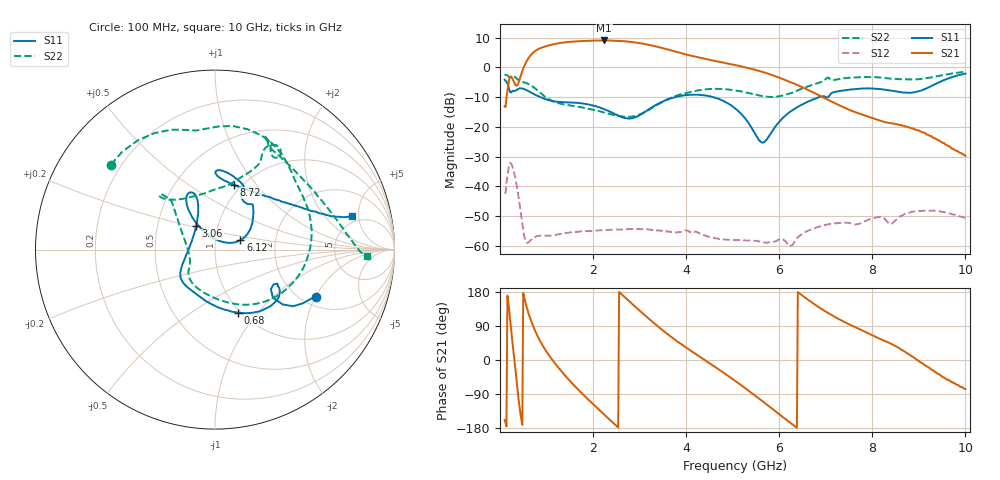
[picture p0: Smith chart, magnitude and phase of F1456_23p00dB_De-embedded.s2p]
! Integrated Device Technology
! Corporate Headquarters
! 6024 Silver Creek Valley Road
! San Jose, CA 95138  USA
! Phone:  1-408-284-8200
! Toll Free:  1-800-223-1366
! Webpage:  http://www.idt.com/
! Timing and RF Division
! 515 Groton Road, Suite 102
! Westford, MA 01886-6024
! Device:  F1456
! Description: 6-bit 0.5 dB Transmit Variable Gain Amplifier
! Frequency:  2100.0 -  2950.00 MHz
! Package:  6x6 mm Thin QFN Plastic Package: 28 pin
! State:  46
! Atten State:  23.0 dB
! Voltage:  +5.00 Volts
! Current:  216.983 mA
! Data:  The device was measured on a the F1455 evaluation board which has
!  individual transmission lines to the RF pins.  Data was collected
!  using a calibrated network analyzer.  The evaluation board was
!  de-embedded using a TRL calibration technique.
!  The reference plane is the edge of the package pin.
!  Pin  1 = CSb
!  Pin  2 = DATA
!  Pin  3 = CLK
!  Pin  4 = RSET
!  Pin  5 = GND
!  Pin  6 = RFIN  = Port 1
!  Pin  7 = GND
!  Pin  8 = NC
!  Pin  9 = NC
!  Pin 10 = NC
!  Pin 11 = NC
!  Pin 12 = NC
!  Pin 13 = NC
!  Pin 14 = /STBY
!  Pin 15 = GND
!  Pin 16 = RFOUT  = Port 2
!  Pin 17 = GND
!  Pin 18 = NC
!  Pin 19 = NC
!  Pin 20 = NC
!  Pin 21 = GND
!  Pin 22 = NC
!  Pin 23 = GND
!  Pin 24 = NC
!  Pin 25 = NC
!  Pin 26 = NC
!  Pin 27 = GND
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# GHz S dB R 50
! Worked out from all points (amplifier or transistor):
!   496 points, 100 MHz to 10 GHz, reference 50 ohm
!   highest |S21| = 9.1 dB at 2.24 GHz (marker M1)
!   |S21| within 3 dB of that: 812.1 MHz to 3.6 GHz (2.788 GHz wide, 126 % of centre)
!   unconditionally stable (mu >= 1): start of sweep to end of sweep
!   at 1.74 GHz: K = 93.20, MAG = 9.3 dB, |S12| = -55.2 dB
!   at 5.06 GHz: K = 294.27, MAG = 1.8 dB, |S12| = -58.1 dB
!   at 10 GHz: K = 578.35, MAG = -20.2 dB, |S12| = -50.7 dB
!   S11 on the Smith chart (normalised r, x): 100 MHz: 2.37, -2.01; 680 MHz: 0.97, -0.79; 3.06 GHz: 0.78, +0.21; 6.12 GHz: 1.32, +0.14; 8.72 GHz: 0.93, +0.78; 10 GHz: 4.18, +4.10
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0.1  -4.15 -24.9  -13.12 -158.1  -42.30 49.6  -2.52 140.8
0.24  -8.42 -30.8  -3.10 79.2  -32.33 -76.2  -3.41 94.4
0.32  -7.88 -29.9  -5.52 -10.6  -36.48 -153.8  -3.27 67.7
0.42  -7.06 -37.0  -4.18 -123.9  -45.80 139.8  -4.58 41.0
0.54  -7.42 -53.7  1.07 155.2  -57.96 132.8  -5.12 15.4
0.68  -8.57 -70.3  4.47 99.9  -57.91 144.1  -6.20 -16.5
0.86  -9.95 -88.5  6.43 50.7  -56.67 112.4  -8.43 -52.9
1.16  -11.42 -113.1  7.82 -5.3  -56.48 77.9  -11.55 -93.2
1.48  -11.76 -130.3  8.57 -52.1  -55.63 54.4  -12.75 -119.4
1.76  -12.11 -140.5  8.87 -87.9  -55.17 38.5  -13.46 -132.7
2.24  -14.07 -156.0  9.07 -144.0  -54.78 17.5  -15.18 -145.6
2.62  -16.74 178.2  8.88 172.8  -54.57 2.2  -16.56 -160.5
3.06  -15.51 128.8  8.02 123.7  -54.43 -18.4  -15.48 166.4
3.4  -12.23 112.4  6.88 88.0  -54.77 -33.4  -12.45 145.6
4.1  -9.20 113.1  3.95 24.5  -55.43 -65.1  -8.25 132.3
5.06  -13.87 125.3  0.78 -55.5  -58.13 -114.5  -7.76 135.6
5.64  -25.33 69.0  -1.52 -108.7  -58.89 -157.4  -9.67 119.1
6.12  -16.39 20.5  -4.21 -154.6  -58.36 166.5  -9.24 85.6
6.7  -10.96 41.3  -8.19 152.0  -54.42 147.9  -5.91 64.0
8.36  -7.70 88.3  -18.71 45.7  -52.62 67.8  -3.75 62.5
8.72  -8.49 73.5  -19.87 20.0  -49.17 68.4  -4.04 50.3
10  -2.10 13.8  -29.78 -76.4  -50.69 -23.5  -1.46 -2.6
